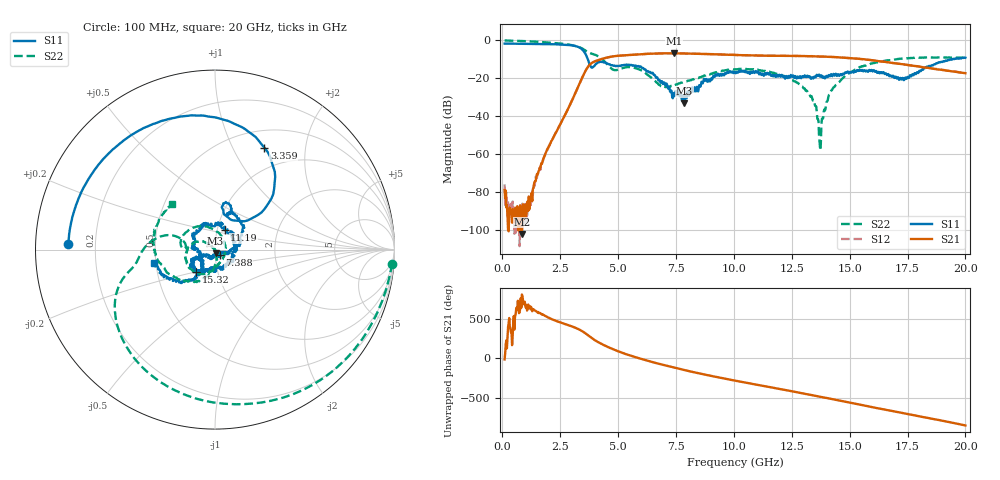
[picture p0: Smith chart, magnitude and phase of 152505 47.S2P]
!  2-Port S-parameters saved by WinCal
! VAR MeasName=S-Parameters (CALIBRATED_DATA) read from VNA (N5230C)
! VAR MeasDate=4/10/2015 9:33:13 AM
! VAR NAME=152505 47
! VAR FILENAME=152505 47.S2P
! VAR DATE=4/10/2015 9:33:13 AM
! VAR PHYS_PORTS=1,2
# Hz S DB R 50
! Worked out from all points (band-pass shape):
!   801 points, 100 MHz to 20 GHz, reference 50 ohm
!   highest |S21| = -6.86 dB at 7.413 GHz (marker M1); lowest = -102.1 dB at 846.2 MHz (marker M2)
!   |S21| within 3 dB of the highest: 4.292 GHz to 15.5 GHz (11.21 GHz wide, 113 % of centre)
!   lowest |S11| = -33.3 dB at 7.861 GHz (marker M3), VSWR 1.04, Z = 50.3 - j2.16 ohm
!   |S11| at or under -10 dB: 3.694 GHz to 19.43 GHz (15.74 GHz wide, 136 % of centre)
!   |S22| runs from -58.0 to -0.1 dB; largest |S21 - S12| = 0.0052
!   S11 on the Smith chart (normalised r, x): 100 MHz: 0.10, +0.02; 3.359 GHz: 0.71, +1.34; 7.388 GHz: 1.05, -0.06; 11.19 GHz: 1.08, +0.24; 15.32 GHz: 0.79, -0.20; 20 GHz: 0.49, -0.08
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1e8  -1.75 177.6  -78.86 -12.3  -75.98 -32.9  -0.09 -4.5
8.4625e8  -1.81 159.7  -102.11 82.5  -90.14 44.8  -0.38 -34.3
1.294e9  -1.88 148.6  -84.82 -126.9  -79.65 -109.4  -0.61 -52.4
2.3885e9  -2.15 116.3  -47.00 104.7  -46.96 104.8  -1.58 -98.5
3.358625e9  -4.00 64.1  -22.21 -2.2  -22.21 -1.8  -3.80 -149.9
3.43325e9  -4.65 57.6  -20.17 -14.3  -20.16 -14.0  -4.23 -154.4
3.856125e9  -14.42 59.1  -12.06 -102.7  -12.08 -102.6  -7.03 -170.4
4.353625e9  -11.52 72.8  -9.63 172.9  -9.65 172.7  -10.40 165.4
5.099875e9  -13.58 69.8  -8.05 79.3  -8.11 79.4  -15.04 177.9
5.92075e9  -13.99 39.1  -7.44 1.6  -7.43 1.8  -15.43 133.1
6.741625e9  -21.15 0.2  -6.93 -65.2  -6.93 -65.4  -23.19 46.6
7.388375e9  -28.12 -50.3  -6.86 -113.0  -6.86 -113.1  -23.77 -42.9
7.41325e9  -27.78 -40.8  -6.86 -114.5  -6.86 -114.5  -23.65 -44.4
7.861e9  -33.27 -81.1  -6.95 -145.4  -6.92 -145.2  -21.98 -74.2
1.005e10  -16.72 135.3  -7.70 81.9  -7.76 81.7  -15.34 -137.6
1.119425e10  -18.28 64.2  -8.05 19.6  -8.10 19.5  -16.09 -175.6
1.338325e10  -19.53 -81.0  -8.43 -100.6  -8.37 -100.4  -30.72 138.5
1.375638e10  -19.04 -93.4  -8.58 -121.9  -8.53 -121.9  -54.71 -90.9
1.420412e10  -17.86 -103.1  -8.80 -147.5  -8.77 -147.9  -26.51 -77.2
1.53235e10  -15.73 -130.4  -9.70 147.9  -9.67 147.1  -14.81 -113.5
1.669162e10  -18.31 -153.0  -11.65 68.8  -11.66 68.4  -10.53 -156.0
2e10  -9.18 -167.9  -17.34 -120.6  -17.29 -120.7  -9.19 133.2
